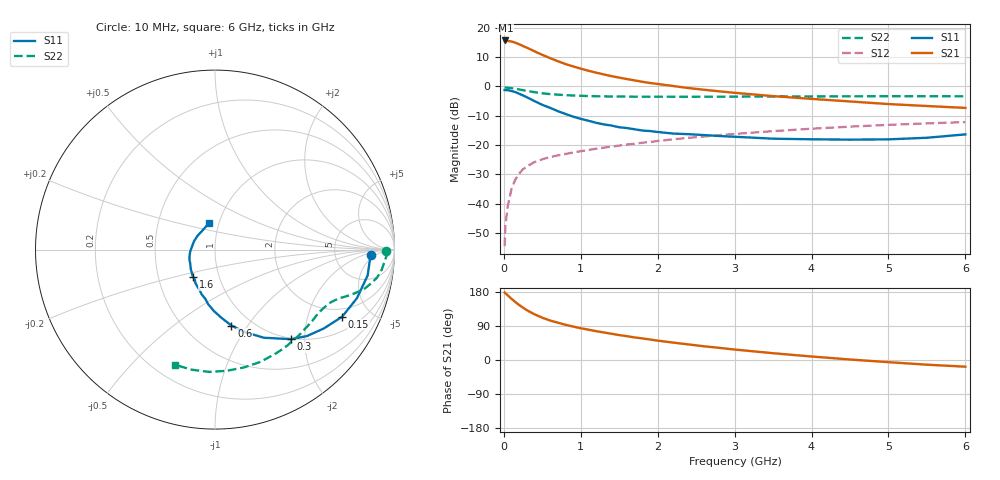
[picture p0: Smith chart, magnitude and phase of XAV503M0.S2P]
! SIEMENS Discrete & RF Semiconductors
! BFY180
! Si NPN RF Bipolar Junction Transistor in MICRO-X
! VCE = 0.5 V  IC = 3 mA
! Common Emitter S-Parameters:  May  1997
# GHz  S  MA  R  50
!  f  S11  S21  S12  S22
! GHz  MAG  ANG  MAG  ANG  MAG  ANG  MAG  ANG
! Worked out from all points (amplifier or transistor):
!   36 points, 10 MHz to 6 GHz, reference 50 ohm
!   highest |S21| = 15.7 dB at 20 MHz (marker M1)
!   |S21| within 3 dB of that: start of sweep to 342.6 MHz
!   unconditionally stable (mu >= 1): start of sweep to 10.19 MHz; 493.5 MHz to end of sweep
!   at 250 MHz: K = 0.57, MSG = 21.0 dB, |S12| = -28.2 dB
!   at 1.4 GHz: K = 1.92, MAG = 6.5 dB, |S12| = -20.5 dB
!   at 6 GHz: K = 2.42, MAG = -4.2 dB, |S12| = -12.1 dB
!   S11 on the Smith chart (normalised r, x): 10 MHz: 14, -3; 150 MHz: 1.60, -3.33; 300 MHz: 0.98, -1.72; 600 MHz: 0.81, -0.84; 1.6 GHz: 0.75, -0.24; 6 GHz: 0.90, +0.27
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0.01  0.8695 -1.9  6.003 178.3  0.0019 85.3  0.9542 -0.5
0.02  0.8647 -3.9  6.075 176.1  0.0042 83.4  0.9596 -1.4
0.05  0.8626 -9.6  5.962 170.7  0.0091 80.1  0.9496 -3.5
0.1  0.8359 -18.9  5.837 161.5  0.018 77.6  0.9354 -6.9
0.15  0.8011 -27.8  5.559 152.9  0.0261 71.7  0.9155 -9.9
0.2  0.749 -35.9  5.226 145.0  0.033 66.3  0.8888 -12.3
0.25  0.7028 -43.3  4.876 138.0  0.0389 61.8  0.8632 -14.5
0.3  0.6542 -49.7  4.573 131.4  0.0434 58.8  0.8394 -16.0
0.4  0.5615 -61.0  3.96 120.4  0.0516 53.6  0.7979 -18.4
0.5  0.4861 -70.5  3.453 111.6  0.0574 50.0  0.7647 -20.2
0.6  0.4329 -77.8  3.04 104.2  0.0626 48.4  0.7406 -21.6
0.8  0.34 -91.4  2.412 92.9  0.0707 46.2  0.7112 -24.2
1  0.2803 -101.0  2.011 83.8  0.0788 45.1  0.6932 -27.0
1.1  0.2603 -106.6  1.848 80.0  0.0826 44.5  0.6865 -28.4
1.4  0.2156 -120.5  1.498 69.2  0.0943 43.8  0.6738 -33.1
1.6  0.1955 -128.8  1.336 62.9  0.1024 43.3  0.672 -36.2
2.2  0.1576 -151.1  1.018 46.0  0.1256 40.7  0.668 -46.3
2.6  0.1486 -163.3  0.879 36.2  0.14 38.1  0.6694 -52.9
3.5  0.1288 171.4  0.684 17.9  0.1732 32.2  0.675 -67.9
4.5  0.1241 142.1  0.555 1.3  0.2067 23.5  0.6786 -84.5
5.5  0.1336 115.2  0.464 -12.4  0.2347 14.6  0.6817 -101.1
6  0.1525 102.2  0.431 -17.6  0.2469 10.1  0.6793 -109.4
